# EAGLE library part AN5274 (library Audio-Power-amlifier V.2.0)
The AN5274 is a monolithic integrated circuit designed for 4.0 W (18 V, 8 W) output audio power amplifier. It is a dual channel SEPP IC suitable for stereo operation in TV application.
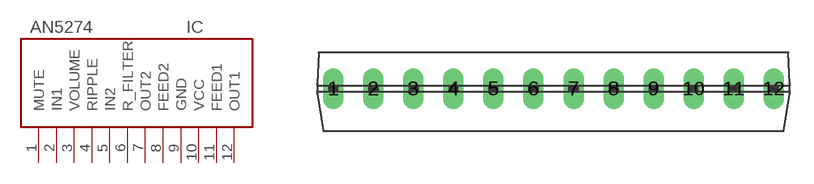
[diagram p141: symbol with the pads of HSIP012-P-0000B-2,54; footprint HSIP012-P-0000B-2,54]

Designator prefix IC

## AN5274  [HSIP012-P-0000B-2,54]
1  MUTE  in
2  IN1  in
3  VOLUME  in
4  RIPPLE
5  IN2  in
6  R_FILTER
7  OUT2  out
8  FEED2
9  GND  pwr
10  VCC  pwr
11  FEED1
12  OUT1  out

## Footprint HSIP012-P-0000B-2,54 (pad centres in mm)
drill 0.8 long: 1 -13.97,0; 2 -11.43,0; 3 -8.89,0; 4 -6.35,0; 5 -3.81,0; 6 -1.27,0; 7 1.27,0; 8 3.81,0; 9 6.35,0; 10 8.89,0; 11 11.43,0; 12 13.97,0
